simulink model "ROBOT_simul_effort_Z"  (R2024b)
settings: Solver=VariableStepAuto  StartTime=0.0  StopTime=5  RelTol=1e-3
undefined symbols (not defined in the file): a, ARRIERE_Defaut_sldprt, avant01_Defaut_sldprt, avant02_Defaut_sldprt, avant03_Defaut_sldprt, avant1_Defaut_sldprt, AXE, BASE_Defaut_sldprt, BIELLE, BIELLE_Defaut_sldprt, BRAS_Defaut_sldprt, bras_Defaut_sldprt, C_Realiste_sldprt, CABLE_Defaut_sldprt, cable_Defaut_sldprt, CACHE_Defaut_sldprt, CARTE, carte_Defaut_sldprt, CARTER, carter, CHC, CODEUR_Defaut_sldprt, cruciforme, cylindrique, deg, Drive, Fichiers, Fichiers_Matlab_sujetA, FIXATION, fixation_Defaut_sldprt, H, HEXAGONALE_Defaut_sldprt, joint_Defaut_sldprt, kg, m, M4, M4_Defaut_sldprt, manette1_Defaut_sldprt, manette2_Defaut_sldprt, MATLAB, Matlab, matlab_Defaut_sldprt, mm, modif, MOTEUR_Defaut_sldprt, N, NEZ_Defaut_sldprt, nom, palier, PARALLELOGRAMME_Defaut_sldprt, petite, plaque, rad, Ressort, Rondelle, ROTOR_Defaut_sldprt, s, SET, simple, socle_Defaut_sldprt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
libraries: sm_lib x463, fl_lib x45, nesl_utility x27, simulink x2
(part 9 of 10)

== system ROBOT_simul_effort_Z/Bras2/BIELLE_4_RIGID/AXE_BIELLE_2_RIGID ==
  ReferenceFrame : sm_lib/Frames and Transforms/Reference Frame
  Solid : sm_lib/Body Elements/File Solid  ExtGeomFileName=/MATLAB Drive/Fichiers_Matlab_sujetA/Fichiers Matlab/STL/AXE BIELLE_Defaut_sldprt.STL  UnitType=Custom  ExtGeomFileUnits=mm  StepReaderType=HEX  ExportConvexHullGeometry=off  InertiaType=Custom  BasedOnType=Density  Density=1000  DensityUnits=kg/(m^3)  Mass=0.0008880235381781051  MassUnits=kg  CenterOfMass=[0 0 0]  CenterOfMassUnits=mm  MomentsOfInertia=[0.018768660222737772 0.018768660222737772 0.0009874025874388381]  MomentsOfInertiaUnits=kg*mm^2  ProductsOfInertia=[0 0 0]  ProductsOfInertiaUnits=kg*mm^2  GraphicType=FromGeometry  MarkerShape=Sphere  MarkerSize=10  GraphicVisPropType=SimpleVisualProperties  GraphicDiffuseColor=[1 0.94901960784313721 0.90980392156862744]  GraphicOpacity=1  GraphicSpecularColor=[0.5 0.5 0.5 1.0]  GraphicAmbientColor=[0.15 0.15 0.15 1.0]  GraphicEmissiveColor=[0.0 0.0 0.0 1.0]  GraphicShininess=75  DoExposeReferenceFrame=on  SerializedFrames=<Frames/>
  F : PMIOPort  Side=Left
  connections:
  Solid/RConn1 -- ReferenceFrame/RConn1 -- F/RConn1

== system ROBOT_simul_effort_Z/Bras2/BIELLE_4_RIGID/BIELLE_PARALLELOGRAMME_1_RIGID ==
  ReferenceFrame : sm_lib/Frames and Transforms/Reference Frame
  Solid : sm_lib/Body Elements/File Solid  ExtGeomFileName=/MATLAB Drive/Fichiers_Matlab_sujetA/Fichiers Matlab/STL/BIELLE PARALLELOGRAMME_Defaut_sldprt.STL  UnitType=Custom  ExtGeomFileUnits=mm  StepReaderType=HEX  ExportConvexHullGeometry=off  InertiaType=Custom  BasedOnType=Density  Density=1000  DensityUnits=kg/(m^3)  Mass=0.0079529027635324764  MassUnits=kg  CenterOfMass=[0 3.1653377955585489 0]  CenterOfMassUnits=mm  MomentsOfInertia=[7.7987017961340088 7.8475939194203406 0.14816857834406802]  MomentsOfInertiaUnits=kg*mm^2  ProductsOfInertia=[0 0 0]  ProductsOfInertiaUnits=kg*mm^2  GraphicType=FromGeometry  MarkerShape=Sphere  MarkerSize=10  GraphicVisPropType=SimpleVisualProperties  GraphicDiffuseColor=[0.6 1.0 1.0]  GraphicOpacity=1  GraphicSpecularColor=[0.5 0.5 0.5 1.0]  GraphicAmbientColor=[0.15 0.15 0.15 1.0]  GraphicEmissiveColor=[0.0 0.0 0.0 1.0]  GraphicShininess=75  DoExposeReferenceFrame=on  SerializedFrames=<Frames/>
  F : PMIOPort  Side=Left
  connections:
  Solid/RConn1 -- ReferenceFrame/RConn1 -- F/RConn1

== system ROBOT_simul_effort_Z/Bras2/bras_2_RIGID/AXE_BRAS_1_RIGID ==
  ReferenceFrame : sm_lib/Frames and Transforms/Reference Frame
  Solid : sm_lib/Body Elements/File Solid  ExtGeomFileName=/MATLAB Drive/Fichiers_Matlab_sujetA/Fichiers Matlab/STL/AXE BRAS_Defaut_sldprt.STL  UnitType=Custom  ExtGeomFileUnits=mm  StepReaderType=HEX  ExportConvexHullGeometry=off  InertiaType=Custom  BasedOnType=Density  Density=1000  DensityUnits=kg/(m^3)  Mass=0.0015327306958088996  MassUnits=kg  CenterOfMass=[0 0 0]  CenterOfMassUnits=mm  MomentsOfInertia=[0.11359646260705632 0.11359646260705632 0.0017137152305883286]  MomentsOfInertiaUnits=kg*mm^2  ProductsOfInertia=[0 0 0]  ProductsOfInertiaUnits=kg*mm^2  GraphicType=FromGeometry  MarkerShape=Sphere  MarkerSize=10  GraphicVisPropType=SimpleVisualProperties  GraphicDiffuseColor=[0.6470588235294118 0.61960784313725492 0.58823529411764708]  GraphicOpacity=1  GraphicSpecularColor=[0.5 0.5 0.5 1.0]  GraphicAmbientColor=[0.15 0.15 0.15 1.0]  GraphicEmissiveColor=[0.0 0.0 0.0 1.0]  GraphicShininess=75  DoExposeReferenceFrame=on  SerializedFrames=<Frames/>
  F : PMIOPort  Side=Left
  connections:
  Solid/RConn1 -- ReferenceFrame/RConn1 -- F/RConn1

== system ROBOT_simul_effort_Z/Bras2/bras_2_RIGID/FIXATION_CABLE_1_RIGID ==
  ReferenceFrame : sm_lib/Frames and Transforms/Reference Frame
  Solid : sm_lib/Body Elements/File Solid  ExtGeomFileName=/MATLAB Drive/Fichiers_Matlab_sujetA/Fichiers Matlab/STL/FIXATION CABLE_Defaut_sldprt.STL  UnitType=Custom  ExtGeomFileUnits=mm  StepReaderType=HEX  ExportConvexHullGeometry=off  InertiaType=Custom  BasedOnType=Density  Density=1000  DensityUnits=kg/(m^3)  Mass=3.2000000000000007e-06  MassUnits=kg  CenterOfMass=[0 0 0.099999999999999992]  CenterOfMassUnits=mm  MomentsOfInertia=[4.2773333333333348e-06 4.2773333333333331e-06 8.5333333333333352e-06]  MomentsOfInertiaUnits=kg*mm^2  ProductsOfInertia=[0 0 0]  ProductsOfInertiaUnits=kg*mm^2  GraphicType=FromGeometry  MarkerShape=Sphere  MarkerSize=10  GraphicVisPropType=SimpleVisualProperties  GraphicDiffuseColor=[0.25098039215686274 0.25098039215686274 0.25098039215686274]  GraphicOpacity=1  GraphicSpecularColor=[0.5 0.5 0.5 1.0]  GraphicAmbientColor=[0.15 0.15 0.15 1.0]  GraphicEmissiveColor=[0.0 0.0 0.0 1.0]  GraphicShininess=75  DoExposeReferenceFrame=on  SerializedFrames=<Frames/>
  F : PMIOPort  Side=Left
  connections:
  Solid/RConn1 -- ReferenceFrame/RConn1 -- F/RConn1

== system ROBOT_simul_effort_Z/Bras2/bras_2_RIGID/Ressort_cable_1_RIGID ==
  ReferenceFrame : sm_lib/Frames and Transforms/Reference Frame
  Solid : sm_lib/Body Elements/File Solid  ExtGeomFileName=/MATLAB Drive/Fichiers_Matlab_sujetA/Fichiers Matlab/STL/Ressort cable_Defaut_sldprt.STL  UnitType=Custom  ExtGeomFileUnits=mm  StepReaderType=HEX  ExportConvexHullGeometry=off  InertiaType=Custom  BasedOnType=Density  Density=1000  DensityUnits=kg/(m^3)  Mass=0.0011765814520035881  MassUnits=kg  CenterOfMass=[0.086849073647483815 -0.00090479521327996976 6.9508776157243597]  CenterOfMassUnits=mm  MomentsOfInertia=[0.034952381374405594 0.034338972761516762 0.0097063586011258158]  MomentsOfInertiaUnits=kg*mm^2  ProductsOfInertia=[0.00037229322226744533 1.6947615167207185e-06 2.0937803976811866e-06]  ProductsOfInertiaUnits=kg*mm^2  GraphicType=FromGeometry  MarkerShape=Sphere  MarkerSize=10  GraphicVisPropType=SimpleVisualProperties  GraphicDiffuseColor=[0.6470588235294118 0.61960784313725492 0.58823529411764708]  GraphicOpacity=1  GraphicSpecularColor=[0.5 0.5 0.5 1.0]  GraphicAmbientColor=[0.15 0.15 0.15 1.0]  GraphicEmissiveColor=[0.0 0.0 0.0 1.0]  GraphicShininess=75  DoExposeReferenceFrame=on  SerializedFrames=<Frames/>
  F : PMIOPort  Side=Left
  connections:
  Solid/RConn1 -- ReferenceFrame/RConn1 -- F/RConn1

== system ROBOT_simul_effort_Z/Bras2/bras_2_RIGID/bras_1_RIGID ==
  ReferenceFrame : sm_lib/Frames and Transforms/Reference Frame
  Solid : sm_lib/Body Elements/File Solid  ExtGeomFileName=/MATLAB Drive/Fichiers_Matlab_sujetA/Fichiers Matlab/STL/bras_Defaut_sldprt.STL  UnitType=Custom  ExtGeomFileUnits=mm  StepReaderType=HEX  ExportConvexHullGeometry=off  InertiaType=Custom  BasedOnType=Density  Density=1000  DensityUnits=kg/(m^3)  Mass=0.06566875822643542  MassUnits=kg  CenterOfMass=[23.925748169887701 -4.7774352723885904 0.0071346362933715022]  CenterOfMassUnits=mm  MomentsOfInertia=[75.153076467382206 23.577652078949701 94.231108050856861]  MomentsOfInertiaUnits=kg*mm^2  ProductsOfInertia=[0.01532312637695204 0.0017211125494294708 -5.8798668472039237]  ProductsOfInertiaUnits=kg*mm^2  GraphicType=FromGeometry  MarkerShape=Sphere  MarkerSize=10  GraphicVisPropType=SimpleVisualProperties  GraphicDiffuseColor=[1.0 1.0 0.0]  GraphicOpacity=1  GraphicSpecularColor=[0.5 0.5 0.5 1.0]  GraphicAmbientColor=[0.15 0.15 0.15 1.0]  GraphicEmissiveColor=[0.0 0.0 0.0 1.0]  GraphicShininess=75  DoExposeReferenceFrame=on  SerializedFrames=<Frames/>
  F : PMIOPort  Side=Left
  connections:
  Solid/RConn1 -- ReferenceFrame/RConn1 -- F/RConn1

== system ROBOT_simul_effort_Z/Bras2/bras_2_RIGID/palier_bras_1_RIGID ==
  ReferenceFrame : sm_lib/Frames and Transforms/Reference Frame
  Solid : sm_lib/Body Elements/File Solid  ExtGeomFileName=/MATLAB Drive/Fichiers_Matlab_sujetA/Fichiers Matlab/STL/palier bras_Defaut_sldprt.STL  UnitType=Custom  ExtGeomFileUnits=mm  StepReaderType=HEX  ExportConvexHullGeometry=off  InertiaType=Custom  BasedOnType=Density  Density=1000  DensityUnits=kg/(m^3)  Mass=0.00017920168094851793  MassUnits=kg  CenterOfMass=[-178.32667601154176 39.825618202078154 -20.980989744703667]  CenterOfMassUnits=mm  MomentsOfInertia=[0.0018602253674838991 0.0012789874237151958 0.0012789874237151961]  MomentsOfInertiaUnits=kg*mm^2  ProductsOfInertia=[0 0 0]  ProductsOfInertiaUnits=kg*mm^2  GraphicType=FromGeometry  MarkerShape=Sphere  MarkerSize=10  GraphicVisPropType=SimpleVisualProperties  GraphicDiffuseColor=[1 1 1]  GraphicOpacity=1  GraphicSpecularColor=[0.5 0.5 0.5 1.0]  GraphicAmbientColor=[0.15 0.15 0.15 1.0]  GraphicEmissiveColor=[0.0 0.0 0.0 1.0]  GraphicShininess=75  DoExposeReferenceFrame=on  SerializedFrames=<Frames/>
  F : PMIOPort  Side=Left
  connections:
  Solid/RConn1 -- ReferenceFrame/RConn1 -- F/RConn1

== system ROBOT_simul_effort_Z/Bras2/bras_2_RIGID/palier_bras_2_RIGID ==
  ReferenceFrame : sm_lib/Frames and Transforms/Reference Frame
  Solid : sm_lib/Body Elements/File Solid  ExtGeomFileName=/MATLAB Drive/Fichiers_Matlab_sujetA/Fichiers Matlab/STL/palier bras_Defaut_sldprt.STL  UnitType=Custom  ExtGeomFileUnits=mm  StepReaderType=HEX  ExportConvexHullGeometry=off  InertiaType=Custom  BasedOnType=Density  Density=1000  DensityUnits=kg/(m^3)  Mass=0.00017920168094851793  MassUnits=kg  CenterOfMass=[-178.32667601154176 39.825618202078154 -20.980989744703667]  CenterOfMassUnits=mm  MomentsOfInertia=[0.0018602253674838991 0.0012789874237151958 0.0012789874237151961]  MomentsOfInertiaUnits=kg*mm^2  ProductsOfInertia=[0 0 0]  ProductsOfInertiaUnits=kg*mm^2  GraphicType=FromGeometry  MarkerShape=Sphere  MarkerSize=10  GraphicVisPropType=SimpleVisualProperties  GraphicDiffuseColor=[1 1 1]  GraphicOpacity=1  GraphicSpecularColor=[0.5 0.5 0.5 1.0]  GraphicAmbientColor=[0.15 0.15 0.15 1.0]  GraphicEmissiveColor=[0.0 0.0 0.0 1.0]  GraphicShininess=75  DoExposeReferenceFrame=on  SerializedFrames=<Frames/>
  F : PMIOPort  Side=Left
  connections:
  Solid/RConn1 -- ReferenceFrame/RConn1 -- F/RConn1

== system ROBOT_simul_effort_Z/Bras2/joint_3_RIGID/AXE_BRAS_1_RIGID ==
  ReferenceFrame : sm_lib/Frames and Transforms/Reference Frame
  Solid : sm_lib/Body Elements/File Solid  ExtGeomFileName=/MATLAB Drive/Fichiers_Matlab_sujetA/Fichiers Matlab/STL/AXE BRAS_Defaut_sldprt.STL  UnitType=Custom  ExtGeomFileUnits=mm  StepReaderType=HEX  ExportConvexHullGeometry=off  InertiaType=Custom  BasedOnType=Density  Density=1000  DensityUnits=kg/(m^3)  Mass=0.0015327306958088996  MassUnits=kg  CenterOfMass=[0 0 0]  CenterOfMassUnits=mm  MomentsOfInertia=[0.11359646260705632 0.11359646260705632 0.0017137152305883286]  MomentsOfInertiaUnits=kg*mm^2  ProductsOfInertia=[0 0 0]  ProductsOfInertiaUnits=kg*mm^2  GraphicType=FromGeometry  MarkerShape=Sphere  MarkerSize=10  GraphicVisPropType=SimpleVisualProperties  GraphicDiffuseColor=[0.6470588235294118 0.61960784313725492 0.58823529411764708]  GraphicOpacity=1  GraphicSpecularColor=[0.5 0.5 0.5 1.0]  GraphicAmbientColor=[0.15 0.15 0.15 1.0]  GraphicEmissiveColor=[0.0 0.0 0.0 1.0]  GraphicShininess=75  DoExposeReferenceFrame=on  SerializedFrames=<Frames/>
  F : PMIOPort  Side=Left
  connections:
  Solid/RConn1 -- ReferenceFrame/RConn1 -- F/RConn1

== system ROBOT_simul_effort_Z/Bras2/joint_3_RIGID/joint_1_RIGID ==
  ReferenceFrame : sm_lib/Frames and Transforms/Reference Frame
  Solid : sm_lib/Body Elements/File Solid  ExtGeomFileName=/MATLAB Drive/Fichiers_Matlab_sujetA/Fichiers Matlab/STL/joint_Defaut_sldprt.STL  UnitType=Custom  ExtGeomFileUnits=mm  StepReaderType=HEX  ExportConvexHullGeometry=off  InertiaType=Custom  BasedOnType=Density  Density=1000  DensityUnits=kg/(m^3)  Mass=0.0062454336323428689  MassUnits=kg  CenterOfMass=[-4.7519597301086606e-06 14.873568128586268 0.2827021501004604]  CenterOfMassUnits=mm  MomentsOfInertia=[0.43544209184236687 0.81590742360241675 0.91424830357082487]  MomentsOfInertiaUnits=kg*mm^2  ProductsOfInertia=[0.0068320776316595647 -4.173068650825101e-06 -7.5142319098046527e-07]  ProductsOfInertiaUnits=kg*mm^2  GraphicType=FromGeometry  MarkerShape=Sphere  MarkerSize=10  GraphicVisPropType=SimpleVisualProperties  GraphicDiffuseColor=[1 1 1]  GraphicOpacity=1  GraphicSpecularColor=[0.5 0.5 0.5 1.0]  GraphicAmbientColor=[0.15 0.15 0.15 1.0]  GraphicEmissiveColor=[0.0 0.0 0.0 1.0]  GraphicShininess=75  DoExposeReferenceFrame=on  SerializedFrames=<Frames/>
  F : PMIOPort  Side=Left
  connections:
  Solid/RConn1 -- ReferenceFrame/RConn1 -- F/RConn1

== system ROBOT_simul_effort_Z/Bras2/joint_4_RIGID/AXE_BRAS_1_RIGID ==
  ReferenceFrame : sm_lib/Frames and Transforms/Reference Frame
  Solid : sm_lib/Body Elements/File Solid  ExtGeomFileName=/MATLAB Drive/Fichiers_Matlab_sujetA/Fichiers Matlab/STL/AXE BRAS_Defaut_sldprt.STL  UnitType=Custom  ExtGeomFileUnits=mm  StepReaderType=HEX  ExportConvexHullGeometry=off  InertiaType=Custom  BasedOnType=Density  Density=1000  DensityUnits=kg/(m^3)  Mass=0.0015327306958088996  MassUnits=kg  CenterOfMass=[0 0 0]  CenterOfMassUnits=mm  MomentsOfInertia=[0.11359646260705632 0.11359646260705632 0.0017137152305883286]  MomentsOfInertiaUnits=kg*mm^2  ProductsOfInertia=[0 0 0]  ProductsOfInertiaUnits=kg*mm^2  GraphicType=FromGeometry  MarkerShape=Sphere  MarkerSize=10  GraphicVisPropType=SimpleVisualProperties  GraphicDiffuseColor=[0.6470588235294118 0.61960784313725492 0.58823529411764708]  GraphicOpacity=1  GraphicSpecularColor=[0.5 0.5 0.5 1.0]  GraphicAmbientColor=[0.15 0.15 0.15 1.0]  GraphicEmissiveColor=[0.0 0.0 0.0 1.0]  GraphicShininess=75  DoExposeReferenceFrame=on  SerializedFrames=<Frames/>
  F : PMIOPort  Side=Left
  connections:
  Solid/RConn1 -- ReferenceFrame/RConn1 -- F/RConn1

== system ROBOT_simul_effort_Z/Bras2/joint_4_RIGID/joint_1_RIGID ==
  ReferenceFrame : sm_lib/Frames and Transforms/Reference Frame
  Solid : sm_lib/Body Elements/File Solid  ExtGeomFileName=/MATLAB Drive/Fichiers_Matlab_sujetA/Fichiers Matlab/STL/joint_Defaut_sldprt.STL  UnitType=Custom  ExtGeomFileUnits=mm  StepReaderType=HEX  ExportConvexHullGeometry=off  InertiaType=Custom  BasedOnType=Density  Density=1000  DensityUnits=kg/(m^3)  Mass=0.0062454336323428689  MassUnits=kg  CenterOfMass=[-4.7519597301086606e-06 14.873568128586268 0.2827021501004604]  CenterOfMassUnits=mm  MomentsOfInertia=[0.43544209184236687 0.81590742360241675 0.91424830357082487]  MomentsOfInertiaUnits=kg*mm^2  ProductsOfInertia=[0.0068320776316595647 -4.173068650825101e-06 -7.5142319098046527e-07]  ProductsOfInertiaUnits=kg*mm^2  GraphicType=FromGeometry  MarkerShape=Sphere  MarkerSize=10  GraphicVisPropType=SimpleVisualProperties  GraphicDiffuseColor=[1 1 1]  GraphicOpacity=1  GraphicSpecularColor=[0.5 0.5 0.5 1.0]  GraphicAmbientColor=[0.15 0.15 0.15 1.0]  GraphicEmissiveColor=[0.0 0.0 0.0 1.0]  GraphicShininess=75  DoExposeReferenceFrame=on  SerializedFrames=<Frames/>
  F : PMIOPort  Side=Left
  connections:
  Solid/RConn1 -- ReferenceFrame/RConn1 -- F/RConn1

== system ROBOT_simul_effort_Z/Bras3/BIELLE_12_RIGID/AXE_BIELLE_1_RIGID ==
  ReferenceFrame : sm_lib/Frames and Transforms/Reference Frame
  Solid : sm_lib/Body Elements/File Solid  ExtGeomFileName=/MATLAB Drive/Fichiers_Matlab_sujetA/Fichiers Matlab/STL/AXE BIELLE_Defaut_sldprt.STL  UnitType=Custom  ExtGeomFileUnits=mm  StepReaderType=HEX  ExportConvexHullGeometry=off  InertiaType=Custom  BasedOnType=Density  Density=1000  DensityUnits=kg/(m^3)  Mass=0.0008880235381781051  MassUnits=kg  CenterOfMass=[0 0 0]  CenterOfMassUnits=mm  MomentsOfInertia=[0.018768660222737772 0.018768660222737772 0.0009874025874388381]  MomentsOfInertiaUnits=kg*mm^2  ProductsOfInertia=[0 0 0]  ProductsOfInertiaUnits=kg*mm^2  GraphicType=FromGeometry  MarkerShape=Sphere  MarkerSize=10  GraphicVisPropType=SimpleVisualProperties  GraphicDiffuseColor=[1 0.94901960784313721 0.90980392156862744]  GraphicOpacity=1  GraphicSpecularColor=[0.5 0.5 0.5 1.0]  GraphicAmbientColor=[0.15 0.15 0.15 1.0]  GraphicEmissiveColor=[0.0 0.0 0.0 1.0]  GraphicShininess=75  DoExposeReferenceFrame=on  SerializedFrames=<Frames/>
  F : PMIOPort  Side=Left
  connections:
  Solid/RConn1 -- ReferenceFrame/RConn1 -- F/RConn1

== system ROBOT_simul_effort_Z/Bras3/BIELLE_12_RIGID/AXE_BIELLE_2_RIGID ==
  ReferenceFrame : sm_lib/Frames and Transforms/Reference Frame
  Solid : sm_lib/Body Elements/File Solid  ExtGeomFileName=/MATLAB Drive/Fichiers_Matlab_sujetA/Fichiers Matlab/STL/AXE BIELLE_Defaut_sldprt.STL  UnitType=Custom  ExtGeomFileUnits=mm  StepReaderType=HEX  ExportConvexHullGeometry=off  InertiaType=Custom  BasedOnType=Density  Density=1000  DensityUnits=kg/(m^3)  Mass=0.0008880235381781051  MassUnits=kg  CenterOfMass=[0 0 0]  CenterOfMassUnits=mm  MomentsOfInertia=[0.018768660222737772 0.018768660222737772 0.0009874025874388381]  MomentsOfInertiaUnits=kg*mm^2  ProductsOfInertia=[0 0 0]  ProductsOfInertiaUnits=kg*mm^2  GraphicType=FromGeometry  MarkerShape=Sphere  MarkerSize=10  GraphicVisPropType=SimpleVisualProperties  GraphicDiffuseColor=[1 0.94901960784313721 0.90980392156862744]  GraphicOpacity=1  GraphicSpecularColor=[0.5 0.5 0.5 1.0]  GraphicAmbientColor=[0.15 0.15 0.15 1.0]  GraphicEmissiveColor=[0.0 0.0 0.0 1.0]  GraphicShininess=75  DoExposeReferenceFrame=on  SerializedFrames=<Frames/>
  F : PMIOPort  Side=Left
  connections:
  Solid/RConn1 -- ReferenceFrame/RConn1 -- F/RConn1

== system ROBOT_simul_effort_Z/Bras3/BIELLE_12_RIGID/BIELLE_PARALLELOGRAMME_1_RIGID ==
  ReferenceFrame : sm_lib/Frames and Transforms/Reference Frame
  Solid : sm_lib/Body Elements/File Solid  ExtGeomFileName=/MATLAB Drive/Fichiers_Matlab_sujetA/Fichiers Matlab/STL/BIELLE PARALLELOGRAMME_Defaut_sldprt.STL  UnitType=Custom  ExtGeomFileUnits=mm  StepReaderType=HEX  ExportConvexHullGeometry=off  InertiaType=Custom  BasedOnType=Density  Density=1000  DensityUnits=kg/(m^3)  Mass=0.0079529027635324764  MassUnits=kg  CenterOfMass=[0 3.1653377955585489 0]  CenterOfMassUnits=mm  MomentsOfInertia=[7.7987017961340088 7.8475939194203406 0.14816857834406802]  MomentsOfInertiaUnits=kg*mm^2  ProductsOfInertia=[0 0 0]  ProductsOfInertiaUnits=kg*mm^2  GraphicType=FromGeometry  MarkerShape=Sphere  MarkerSize=10  GraphicVisPropType=SimpleVisualProperties  GraphicDiffuseColor=[0.6 1.0 1.0]  GraphicOpacity=1  GraphicSpecularColor=[0.5 0.5 0.5 1.0]  GraphicAmbientColor=[0.15 0.15 0.15 1.0]  GraphicEmissiveColor=[0.0 0.0 0.0 1.0]  GraphicShininess=75  DoExposeReferenceFrame=on  SerializedFrames=<Frames/>
  F : PMIOPort  Side=Left
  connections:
  Solid/RConn1 -- ReferenceFrame/RConn1 -- F/RConn1

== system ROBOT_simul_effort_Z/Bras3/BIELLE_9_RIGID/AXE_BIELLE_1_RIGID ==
  ReferenceFrame : sm_lib/Frames and Transforms/Reference Frame
  Solid : sm_lib/Body Elements/File Solid  ExtGeomFileName=/MATLAB Drive/Fichiers_Matlab_sujetA/Fichiers Matlab/STL/AXE BIELLE_Defaut_sldprt.STL  UnitType=Custom  ExtGeomFileUnits=mm  StepReaderType=HEX  ExportConvexHullGeometry=off  InertiaType=Custom  BasedOnType=Density  Density=1000  DensityUnits=kg/(m^3)  Mass=0.0008880235381781051  MassUnits=kg  CenterOfMass=[0 0 0]  CenterOfMassUnits=mm  MomentsOfInertia=[0.018768660222737772 0.018768660222737772 0.0009874025874388381]  MomentsOfInertiaUnits=kg*mm^2  ProductsOfInertia=[0 0 0]  ProductsOfInertiaUnits=kg*mm^2  GraphicType=FromGeometry  MarkerShape=Sphere  MarkerSize=10  GraphicVisPropType=SimpleVisualProperties  GraphicDiffuseColor=[1 0.94901960784313721 0.90980392156862744]  GraphicOpacity=1  GraphicSpecularColor=[0.5 0.5 0.5 1.0]  GraphicAmbientColor=[0.15 0.15 0.15 1.0]  GraphicEmissiveColor=[0.0 0.0 0.0 1.0]  GraphicShininess=75  DoExposeReferenceFrame=on  SerializedFrames=<Frames/>
  F : PMIOPort  Side=Left
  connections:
  Solid/RConn1 -- ReferenceFrame/RConn1 -- F/RConn1

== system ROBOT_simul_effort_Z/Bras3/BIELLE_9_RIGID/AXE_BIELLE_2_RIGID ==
  ReferenceFrame : sm_lib/Frames and Transforms/Reference Frame
  Solid : sm_lib/Body Elements/File Solid  ExtGeomFileName=/MATLAB Drive/Fichiers_Matlab_sujetA/Fichiers Matlab/STL/AXE BIELLE_Defaut_sldprt.STL  UnitType=Custom  ExtGeomFileUnits=mm  StepReaderType=HEX  ExportConvexHullGeometry=off  InertiaType=Custom  BasedOnType=Density  Density=1000  DensityUnits=kg/(m^3)  Mass=0.0008880235381781051  MassUnits=kg  CenterOfMass=[0 0 0]  CenterOfMassUnits=mm  MomentsOfInertia=[0.018768660222737772 0.018768660222737772 0.0009874025874388381]  MomentsOfInertiaUnits=kg*mm^2  ProductsOfInertia=[0 0 0]  ProductsOfInertiaUnits=kg*mm^2  GraphicType=FromGeometry  MarkerShape=Sphere  MarkerSize=10  GraphicVisPropType=SimpleVisualProperties  GraphicDiffuseColor=[1 0.94901960784313721 0.90980392156862744]  GraphicOpacity=1  GraphicSpecularColor=[0.5 0.5 0.5 1.0]  GraphicAmbientColor=[0.15 0.15 0.15 1.0]  GraphicEmissiveColor=[0.0 0.0 0.0 1.0]  GraphicShininess=75  DoExposeReferenceFrame=on  SerializedFrames=<Frames/>
  F : PMIOPort  Side=Left
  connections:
  Solid/RConn1 -- ReferenceFrame/RConn1 -- F/RConn1

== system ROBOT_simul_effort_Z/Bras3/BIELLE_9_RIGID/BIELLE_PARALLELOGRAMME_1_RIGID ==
  ReferenceFrame : sm_lib/Frames and Transforms/Reference Frame
  Solid : sm_lib/Body Elements/File Solid  ExtGeomFileName=/MATLAB Drive/Fichiers_Matlab_sujetA/Fichiers Matlab/STL/BIELLE PARALLELOGRAMME_Defaut_sldprt.STL  UnitType=Custom  ExtGeomFileUnits=mm  StepReaderType=HEX  ExportConvexHullGeometry=off  InertiaType=Custom  BasedOnType=Density  Density=1000  DensityUnits=kg/(m^3)  Mass=0.0079529027635324764  MassUnits=kg  CenterOfMass=[0 3.1653377955585489 0]  CenterOfMassUnits=mm  MomentsOfInertia=[7.7987017961340088 7.8475939194203406 0.14816857834406802]  MomentsOfInertiaUnits=kg*mm^2  ProductsOfInertia=[0 0 0]  ProductsOfInertiaUnits=kg*mm^2  GraphicType=FromGeometry  MarkerShape=Sphere  MarkerSize=10  GraphicVisPropType=SimpleVisualProperties  GraphicDiffuseColor=[0.6 1.0 1.0]  GraphicOpacity=1  GraphicSpecularColor=[0.5 0.5 0.5 1.0]  GraphicAmbientColor=[0.15 0.15 0.15 1.0]  GraphicEmissiveColor=[0.0 0.0 0.0 1.0]  GraphicShininess=75  DoExposeReferenceFrame=on  SerializedFrames=<Frames/>
  F : PMIOPort  Side=Left
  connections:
  Solid/RConn1 -- ReferenceFrame/RConn1 -- F/RConn1

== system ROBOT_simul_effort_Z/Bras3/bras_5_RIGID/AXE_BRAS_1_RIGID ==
  ReferenceFrame : sm_lib/Frames and Transforms/Reference Frame
  Solid : sm_lib/Body Elements/File Solid  ExtGeomFileName=/MATLAB Drive/Fichiers_Matlab_sujetA/Fichiers Matlab/STL/AXE BRAS_Defaut_sldprt.STL  UnitType=Custom  ExtGeomFileUnits=mm  StepReaderType=HEX  ExportConvexHullGeometry=off  InertiaType=Custom  BasedOnType=Density  Density=1000  DensityUnits=kg/(m^3)  Mass=0.0015327306958088996  MassUnits=kg  CenterOfMass=[0 0 0]  CenterOfMassUnits=mm  MomentsOfInertia=[0.11359646260705632 0.11359646260705632 0.0017137152305883286]  MomentsOfInertiaUnits=kg*mm^2  ProductsOfInertia=[0 0 0]  ProductsOfInertiaUnits=kg*mm^2  GraphicType=FromGeometry  MarkerShape=Sphere  MarkerSize=10  GraphicVisPropType=SimpleVisualProperties  GraphicDiffuseColor=[0.6470588235294118 0.61960784313725492 0.58823529411764708]  GraphicOpacity=1  GraphicSpecularColor=[0.5 0.5 0.5 1.0]  GraphicAmbientColor=[0.15 0.15 0.15 1.0]  GraphicEmissiveColor=[0.0 0.0 0.0 1.0]  GraphicShininess=75  DoExposeReferenceFrame=on  SerializedFrames=<Frames/>
  F : PMIOPort  Side=Left
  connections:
  Solid/RConn1 -- ReferenceFrame/RConn1 -- F/RConn1

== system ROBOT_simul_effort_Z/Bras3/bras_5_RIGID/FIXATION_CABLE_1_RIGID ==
  ReferenceFrame : sm_lib/Frames and Transforms/Reference Frame
  Solid : sm_lib/Body Elements/File Solid  ExtGeomFileName=/MATLAB Drive/Fichiers_Matlab_sujetA/Fichiers Matlab/STL/FIXATION CABLE_Defaut_sldprt.STL  UnitType=Custom  ExtGeomFileUnits=mm  StepReaderType=HEX  ExportConvexHullGeometry=off  InertiaType=Custom  BasedOnType=Density  Density=1000  DensityUnits=kg/(m^3)  Mass=3.2000000000000007e-06  MassUnits=kg  CenterOfMass=[0 0 0.099999999999999992]  CenterOfMassUnits=mm  MomentsOfInertia=[4.2773333333333348e-06 4.2773333333333331e-06 8.5333333333333352e-06]  MomentsOfInertiaUnits=kg*mm^2  ProductsOfInertia=[0 0 0]  ProductsOfInertiaUnits=kg*mm^2  GraphicType=FromGeometry  MarkerShape=Sphere  MarkerSize=10  GraphicVisPropType=SimpleVisualProperties  GraphicDiffuseColor=[0.25098039215686274 0.25098039215686274 0.25098039215686274]  GraphicOpacity=1  GraphicSpecularColor=[0.5 0.5 0.5 1.0]  GraphicAmbientColor=[0.15 0.15 0.15 1.0]  GraphicEmissiveColor=[0.0 0.0 0.0 1.0]  GraphicShininess=75  DoExposeReferenceFrame=on  SerializedFrames=<Frames/>
  F : PMIOPort  Side=Left
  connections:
  Solid/RConn1 -- ReferenceFrame/RConn1 -- F/RConn1

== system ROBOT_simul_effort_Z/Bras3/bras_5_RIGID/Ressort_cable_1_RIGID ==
  ReferenceFrame : sm_lib/Frames and Transforms/Reference Frame
  Solid : sm_lib/Body Elements/File Solid  ExtGeomFileName=/MATLAB Drive/Fichiers_Matlab_sujetA/Fichiers Matlab/STL/Ressort cable_Defaut_sldprt.STL  UnitType=Custom  ExtGeomFileUnits=mm  StepReaderType=HEX  ExportConvexHullGeometry=off  InertiaType=Custom  BasedOnType=Density  Density=1000  DensityUnits=kg/(m^3)  Mass=0.0011765814520035881  MassUnits=kg  CenterOfMass=[0.086849073647483815 -0.00090479521327996976 6.9508776157243597]  CenterOfMassUnits=mm  MomentsOfInertia=[0.034952381374405594 0.034338972761516762 0.0097063586011258158]  MomentsOfInertiaUnits=kg*mm^2  ProductsOfInertia=[0.00037229322226744533 1.6947615167207185e-06 2.0937803976811866e-06]  ProductsOfInertiaUnits=kg*mm^2  GraphicType=FromGeometry  MarkerShape=Sphere  MarkerSize=10  GraphicVisPropType=SimpleVisualProperties  GraphicDiffuseColor=[0.6470588235294118 0.61960784313725492 0.58823529411764708]  GraphicOpacity=1  GraphicSpecularColor=[0.5 0.5 0.5 1.0]  GraphicAmbientColor=[0.15 0.15 0.15 1.0]  GraphicEmissiveColor=[0.0 0.0 0.0 1.0]  GraphicShininess=75  DoExposeReferenceFrame=on  SerializedFrames=<Frames/>
  F : PMIOPort  Side=Left
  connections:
  Solid/RConn1 -- ReferenceFrame/RConn1 -- F/RConn1

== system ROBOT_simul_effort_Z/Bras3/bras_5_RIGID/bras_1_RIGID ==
  ReferenceFrame : sm_lib/Frames and Transforms/Reference Frame
  Solid : sm_lib/Body Elements/File Solid  ExtGeomFileName=/MATLAB Drive/Fichiers_Matlab_sujetA/Fichiers Matlab/STL/bras_Defaut_sldprt.STL  UnitType=Custom  ExtGeomFileUnits=mm  StepReaderType=HEX  ExportConvexHullGeometry=off  InertiaType=Custom  BasedOnType=Density  Density=1000  DensityUnits=kg/(m^3)  Mass=0.06566875822643542  MassUnits=kg  CenterOfMass=[23.925748169887701 -4.7774352723885904 0.0071346362933715022]  CenterOfMassUnits=mm  MomentsOfInertia=[75.153076467382206 23.577652078949701 94.231108050856861]  MomentsOfInertiaUnits=kg*mm^2  ProductsOfInertia=[0.01532312637695204 0.0017211125494294708 -5.8798668472039237]  ProductsOfInertiaUnits=kg*mm^2  GraphicType=FromGeometry  MarkerShape=Sphere  MarkerSize=10  GraphicVisPropType=SimpleVisualProperties  GraphicDiffuseColor=[1.0 1.0 0.0]  GraphicOpacity=1  GraphicSpecularColor=[0.5 0.5 0.5 1.0]  GraphicAmbientColor=[0.15 0.15 0.15 1.0]  GraphicEmissiveColor=[0.0 0.0 0.0 1.0]  GraphicShininess=75  DoExposeReferenceFrame=on  SerializedFrames=<Frames/>
  F : PMIOPort  Side=Left
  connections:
  Solid/RConn1 -- ReferenceFrame/RConn1 -- F/RConn1

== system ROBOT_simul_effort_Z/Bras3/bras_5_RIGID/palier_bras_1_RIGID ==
  ReferenceFrame : sm_lib/Frames and Transforms/Reference Frame
  Solid : sm_lib/Body Elements/File Solid  ExtGeomFileName=/MATLAB Drive/Fichiers_Matlab_sujetA/Fichiers Matlab/STL/palier bras_Defaut_sldprt.STL  UnitType=Custom  ExtGeomFileUnits=mm  StepReaderType=HEX  ExportConvexHullGeometry=off  InertiaType=Custom  BasedOnType=Density  Density=1000  DensityUnits=kg/(m^3)  Mass=0.00017920168094851793  MassUnits=kg  CenterOfMass=[-178.32667601154176 39.825618202078154 -20.980989744703667]  CenterOfMassUnits=mm  MomentsOfInertia=[0.0018602253674838991 0.0012789874237151958 0.0012789874237151961]  MomentsOfInertiaUnits=kg*mm^2  ProductsOfInertia=[0 0 0]  ProductsOfInertiaUnits=kg*mm^2  GraphicType=FromGeometry  MarkerShape=Sphere  MarkerSize=10  GraphicVisPropType=SimpleVisualProperties  GraphicDiffuseColor=[1 1 1]  GraphicOpacity=1  GraphicSpecularColor=[0.5 0.5 0.5 1.0]  GraphicAmbientColor=[0.15 0.15 0.15 1.0]  GraphicEmissiveColor=[0.0 0.0 0.0 1.0]  GraphicShininess=75  DoExposeReferenceFrame=on  SerializedFrames=<Frames/>
  F : PMIOPort  Side=Left
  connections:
  Solid/RConn1 -- ReferenceFrame/RConn1 -- F/RConn1

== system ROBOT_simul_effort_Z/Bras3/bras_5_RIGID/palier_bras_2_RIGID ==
  ReferenceFrame : sm_lib/Frames and Transforms/Reference Frame
  Solid : sm_lib/Body Elements/File Solid  ExtGeomFileName=/MATLAB Drive/Fichiers_Matlab_sujetA/Fichiers Matlab/STL/palier bras_Defaut_sldprt.STL  UnitType=Custom  ExtGeomFileUnits=mm  StepReaderType=HEX  ExportConvexHullGeometry=off  InertiaType=Custom  BasedOnType=Density  Density=1000  DensityUnits=kg/(m^3)  Mass=0.00017920168094851793  MassUnits=kg  CenterOfMass=[-178.32667601154176 39.825618202078154 -20.980989744703667]  CenterOfMassUnits=mm  MomentsOfInertia=[0.0018602253674838991 0.0012789874237151958 0.0012789874237151961]  MomentsOfInertiaUnits=kg*mm^2  ProductsOfInertia=[0 0 0]  ProductsOfInertiaUnits=kg*mm^2  GraphicType=FromGeometry  MarkerShape=Sphere  MarkerSize=10  GraphicVisPropType=SimpleVisualProperties  GraphicDiffuseColor=[1 1 1]  GraphicOpacity=1  GraphicSpecularColor=[0.5 0.5 0.5 1.0]  GraphicAmbientColor=[0.15 0.15 0.15 1.0]  GraphicEmissiveColor=[0.0 0.0 0.0 1.0]  GraphicShininess=75  DoExposeReferenceFrame=on  SerializedFrames=<Frames/>
  F : PMIOPort  Side=Left
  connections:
  Solid/RConn1 -- ReferenceFrame/RConn1 -- F/RConn1

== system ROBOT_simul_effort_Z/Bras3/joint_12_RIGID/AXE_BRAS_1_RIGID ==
  ReferenceFrame : sm_lib/Frames and Transforms/Reference Frame
  Solid : sm_lib/Body Elements/File Solid  ExtGeomFileName=/MATLAB Drive/Fichiers_Matlab_sujetA/Fichiers Matlab/STL/AXE BRAS_Defaut_sldprt.STL  UnitType=Custom  ExtGeomFileUnits=mm  StepReaderType=HEX  ExportConvexHullGeometry=off  InertiaType=Custom  BasedOnType=Density  Density=1000  DensityUnits=kg/(m^3)  Mass=0.0015327306958088996  MassUnits=kg  CenterOfMass=[0 0 0]  CenterOfMassUnits=mm  MomentsOfInertia=[0.11359646260705632 0.11359646260705632 0.0017137152305883286]  MomentsOfInertiaUnits=kg*mm^2  ProductsOfInertia=[0 0 0]  ProductsOfInertiaUnits=kg*mm^2  GraphicType=FromGeometry  MarkerShape=Sphere  MarkerSize=10  GraphicVisPropType=SimpleVisualProperties  GraphicDiffuseColor=[0.6470588235294118 0.61960784313725492 0.58823529411764708]  GraphicOpacity=1  GraphicSpecularColor=[0.5 0.5 0.5 1.0]  GraphicAmbientColor=[0.15 0.15 0.15 1.0]  GraphicEmissiveColor=[0.0 0.0 0.0 1.0]  GraphicShininess=75  DoExposeReferenceFrame=on  SerializedFrames=<Frames/>
  F : PMIOPort  Side=Left
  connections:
  Solid/RConn1 -- ReferenceFrame/RConn1 -- F/RConn1

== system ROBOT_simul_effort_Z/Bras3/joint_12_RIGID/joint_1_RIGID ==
  ReferenceFrame : sm_lib/Frames and Transforms/Reference Frame
  Solid : sm_lib/Body Elements/File Solid  ExtGeomFileName=/MATLAB Drive/Fichiers_Matlab_sujetA/Fichiers Matlab/STL/joint_Defaut_sldprt.STL  UnitType=Custom  ExtGeomFileUnits=mm  StepReaderType=HEX  ExportConvexHullGeometry=off  InertiaType=Custom  BasedOnType=Density  Density=1000  DensityUnits=kg/(m^3)  Mass=0.0062454336323428689  MassUnits=kg  CenterOfMass=[-4.7519597301086606e-06 14.873568128586268 0.2827021501004604]  CenterOfMassUnits=mm  MomentsOfInertia=[0.43544209184236687 0.81590742360241675 0.91424830357082487]  MomentsOfInertiaUnits=kg*mm^2  ProductsOfInertia=[0.0068320776316595647 -4.173068650825101e-06 -7.5142319098046527e-07]  ProductsOfInertiaUnits=kg*mm^2  GraphicType=FromGeometry  MarkerShape=Sphere  MarkerSize=10  GraphicVisPropType=SimpleVisualProperties  GraphicDiffuseColor=[1 1 1]  GraphicOpacity=1  GraphicSpecularColor=[0.5 0.5 0.5 1.0]  GraphicAmbientColor=[0.15 0.15 0.15 1.0]  GraphicEmissiveColor=[0.0 0.0 0.0 1.0]  GraphicShininess=75  DoExposeReferenceFrame=on  SerializedFrames=<Frames/>
  F : PMIOPort  Side=Left
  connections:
  Solid/RConn1 -- ReferenceFrame/RConn1 -- F/RConn1

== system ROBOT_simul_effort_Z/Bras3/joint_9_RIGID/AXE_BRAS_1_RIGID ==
  ReferenceFrame : sm_lib/Frames and Transforms/Reference Frame
  Solid : sm_lib/Body Elements/File Solid  ExtGeomFileName=/MATLAB Drive/Fichiers_Matlab_sujetA/Fichiers Matlab/STL/AXE BRAS_Defaut_sldprt.STL  UnitType=Custom  ExtGeomFileUnits=mm  StepReaderType=HEX  ExportConvexHullGeometry=off  InertiaType=Custom  BasedOnType=Density  Density=1000  DensityUnits=kg/(m^3)  Mass=0.0015327306958088996  MassUnits=kg  CenterOfMass=[0 0 0]  CenterOfMassUnits=mm  MomentsOfInertia=[0.11359646260705632 0.11359646260705632 0.0017137152305883286]  MomentsOfInertiaUnits=kg*mm^2  ProductsOfInertia=[0 0 0]  ProductsOfInertiaUnits=kg*mm^2  GraphicType=FromGeometry  MarkerShape=Sphere  MarkerSize=10  GraphicVisPropType=SimpleVisualProperties  GraphicDiffuseColor=[0.6470588235294118 0.61960784313725492 0.58823529411764708]  GraphicOpacity=1  GraphicSpecularColor=[0.5 0.5 0.5 1.0]  GraphicAmbientColor=[0.15 0.15 0.15 1.0]  GraphicEmissiveColor=[0.0 0.0 0.0 1.0]  GraphicShininess=75  DoExposeReferenceFrame=on  SerializedFrames=<Frames/>
  F : PMIOPort  Side=Left
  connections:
  Solid/RConn1 -- ReferenceFrame/RConn1 -- F/RConn1

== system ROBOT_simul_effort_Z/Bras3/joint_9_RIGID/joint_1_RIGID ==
  ReferenceFrame : sm_lib/Frames and Transforms/Reference Frame
  Solid : sm_lib/Body Elements/File Solid  ExtGeomFileName=/MATLAB Drive/Fichiers_Matlab_sujetA/Fichiers Matlab/STL/joint_Defaut_sldprt.STL  UnitType=Custom  ExtGeomFileUnits=mm  StepReaderType=HEX  ExportConvexHullGeometry=off  InertiaType=Custom  BasedOnType=Density  Density=1000  DensityUnits=kg/(m^3)  Mass=0.0062454336323428689  MassUnits=kg  CenterOfMass=[-4.7519597301086606e-06 14.873568128586268 0.2827021501004604]  CenterOfMassUnits=mm  MomentsOfInertia=[0.43544209184236687 0.81590742360241675 0.91424830357082487]  MomentsOfInertiaUnits=kg*mm^2  ProductsOfInertia=[0.0068320776316595647 -4.173068650825101e-06 -7.5142319098046527e-07]  ProductsOfInertiaUnits=kg*mm^2  GraphicType=FromGeometry  MarkerShape=Sphere  MarkerSize=10  GraphicVisPropType=SimpleVisualProperties  GraphicDiffuseColor=[1 1 1]  GraphicOpacity=1  GraphicSpecularColor=[0.5 0.5 0.5 1.0]  GraphicAmbientColor=[0.15 0.15 0.15 1.0]  GraphicEmissiveColor=[0.0 0.0 0.0 1.0]  GraphicShininess=75  DoExposeReferenceFrame=on  SerializedFrames=<Frames/>
  F : PMIOPort  Side=Left
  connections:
  Solid/RConn1 -- ReferenceFrame/RConn1 -- F/RConn1

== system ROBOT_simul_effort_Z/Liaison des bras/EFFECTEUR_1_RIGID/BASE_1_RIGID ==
  ReferenceFrame : sm_lib/Frames and Transforms/Reference Frame
  Solid : sm_lib/Body Elements/File Solid  ExtGeomFileName=/MATLAB Drive/Fichiers_Matlab_sujetA/Fichiers Matlab/STL/BASE_Defaut_sldprt.STL  UnitType=Custom  ExtGeomFileUnits=mm  StepReaderType=HEX  ExportConvexHullGeometry=off  InertiaType=Custom  BasedOnType=Density  Density=1000  DensityUnits=kg/(m^3)  Mass=0.028238598075005058  MassUnits=kg  CenterOfMass=[-0.50940754911928388 -1.6318221689243708 -4.5607511741024656]  CenterOfMassUnits=mm  MomentsOfInertia=[8.5842414198569479 7.5819347196129669 14.129620619032369]  MomentsOfInertiaUnits=kg*mm^2  ProductsOfInertia=[-0.29549774773685261 -0.082418003511546406 -0.14811223553088118]  ProductsOfInertiaUnits=kg*mm^2  GraphicType=FromGeometry  MarkerShape=Sphere  MarkerSize=10  GraphicVisPropType=SimpleVisualProperties  GraphicDiffuseColor=[1.0 1.0 1.0]  GraphicOpacity=1  GraphicSpecularColor=[0.5 0.5 0.5 1.0]  GraphicAmbientColor=[0.15 0.15 0.15 1.0]  GraphicEmissiveColor=[0.0 0.0 0.0 1.0]  GraphicShininess=75  DoExposeReferenceFrame=on  SerializedFrames=<Frames/>
  F : PMIOPort  Side=Left
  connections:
  Solid/RConn1 -- ReferenceFrame/RConn1 -- F/RConn1

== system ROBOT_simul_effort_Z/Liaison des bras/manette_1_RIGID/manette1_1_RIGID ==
  ReferenceFrame : sm_lib/Frames and Transforms/Reference Frame
  Solid : sm_lib/Body Elements/File Solid  ExtGeomFileName=/MATLAB Drive/Fichiers_Matlab_sujetA/Fichiers Matlab/STL/manette1_Defaut_sldprt.STL  UnitType=Custom  ExtGeomFileUnits=mm  StepReaderType=HEX  ExportConvexHullGeometry=off  InertiaType=Custom  BasedOnType=Density  Density=1000  DensityUnits=kg/(m^3)  Mass=0.021495200046783486  MassUnits=kg  CenterOfMass=[-1.4897475291331288 1.1324325333899619 3.6124835128376875]  CenterOfMassUnits=mm  MomentsOfInertia=[5.4184345928892519 5.4614392106741905 10.048915162120133]  MomentsOfInertiaUnits=kg*mm^2  ProductsOfInertia=[-0.010452851512005331 -0.0018797921399214363 0.024517118393881449]  ProductsOfInertiaUnits=kg*mm^2  GraphicType=FromGeometry  MarkerShape=Sphere  MarkerSize=10  GraphicVisPropType=SimpleVisualProperties  GraphicDiffuseColor=[0.8 0.8 0.8]  GraphicOpacity=1  GraphicSpecularColor=[0.5 0.5 0.5 1.0]  GraphicAmbientColor=[0.15 0.15 0.15 1.0]  GraphicEmissiveColor=[0.0 0.0 0.0 1.0]  GraphicShininess=75  DoExposeReferenceFrame=on  SerializedFrames=<Frames/>
  F : PMIOPort  Side=Left
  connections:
  Solid/RConn1 -- ReferenceFrame/RConn1 -- F/RConn1

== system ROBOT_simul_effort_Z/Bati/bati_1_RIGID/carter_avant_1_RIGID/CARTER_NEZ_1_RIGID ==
  ReferenceFrame : sm_lib/Frames and Transforms/Reference Frame
  Solid : sm_lib/Body Elements/File Solid  ExtGeomFileName=/MATLAB Drive/Fichiers_Matlab_sujetA/Fichiers Matlab/STL/CARTER NEZ_Defaut_sldprt.STL  UnitType=Custom  ExtGeomFileUnits=mm  StepReaderType=HEX  ExportConvexHullGeometry=off  InertiaType=Custom  BasedOnType=Density  Density=1000  DensityUnits=kg/(m^3)  Mass=0.023684568109850399  MassUnits=kg  CenterOfMass=[17.102684932647009 114.0476537917955 1.3404873933864438]  CenterOfMassUnits=mm  MomentsOfInertia=[16.43130676036915 32.571595129912247 16.431105891514132]  MomentsOfInertiaUnits=kg*mm^2  ProductsOfInertia=[-3.788014627850142e-05 -4.8452777139477129e-05 -5.4026210558728518e-06]  ProductsOfInertiaUnits=kg*mm^2  GraphicType=FromGeometry  MarkerShape=Sphere  MarkerSize=10  GraphicVisPropType=SimpleVisualProperties  GraphicDiffuseColor=[0.75294117647058822 0.75294117647058822 0.75294117647058822]  GraphicOpacity=1  GraphicSpecularColor=[0.5 0.5 0.5 1.0]  GraphicAmbientColor=[0.15 0.15 0.15 1.0]  GraphicEmissiveColor=[0.0 0.0 0.0 1.0]  GraphicShininess=75  DoExposeReferenceFrame=on  SerializedFrames=<Frames/>
  F : PMIOPort  Side=Left
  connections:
  Solid/RConn1 -- ReferenceFrame/RConn1 -- F/RConn1

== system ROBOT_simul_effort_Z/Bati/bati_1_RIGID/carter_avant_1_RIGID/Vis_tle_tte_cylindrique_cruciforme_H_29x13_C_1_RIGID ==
  ReferenceFrame : sm_lib/Frames and Transforms/Reference Frame
  Solid : sm_lib/Body Elements/File Solid  ExtGeomFileName=/MATLAB Drive/Fichiers_Matlab_sujetA/Fichiers Matlab/STL/Vis a tole tete cylindrique cruciforme H 2-9x13 - C_Realiste_sldprt.STL  UnitType=Custom  ExtGeomFileUnits=mm  StepReaderType=HEX  ExportConvexHullGeometry=off  InertiaType=Custom  BasedOnType=Density  Density=1000  DensityUnits=kg/(m^3)  Mass=8.3821869835456372e-05  MassUnits=kg  CenterOfMass=[4.9478681581074904 0.00064910481891303923 -0.0013634218224953438]  CenterOfMassUnits=mm  MomentsOfInertia=[0.00016543197172893975 0.0014334630955093895 0.0014333390308476422]  MomentsOfInertiaUnits=kg*mm^2  ProductsOfInertia=[-5.4062904633677868e-09 -1.3111174919527308e-07 6.0713893531177014e-07]  ProductsOfInertiaUnits=kg*mm^2  GraphicType=FromGeometry  MarkerShape=Sphere  MarkerSize=10  GraphicVisPropType=SimpleVisualProperties  GraphicDiffuseColor=[0.75294117647058822 0.75294117647058822 0.75294117647058822]  GraphicOpacity=1  GraphicSpecularColor=[0.5 0.5 0.5 1.0]  GraphicAmbientColor=[0.15 0.15 0.15 1.0]  GraphicEmissiveColor=[0.0 0.0 0.0 1.0]  GraphicShininess=75  DoExposeReferenceFrame=on  SerializedFrames=<Frames/>
  F : PMIOPort  Side=Left
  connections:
  Solid/RConn1 -- ReferenceFrame/RConn1 -- F/RConn1

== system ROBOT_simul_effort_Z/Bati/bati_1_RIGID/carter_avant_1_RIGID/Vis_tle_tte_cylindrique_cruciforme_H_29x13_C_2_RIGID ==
  ReferenceFrame : sm_lib/Frames and Transforms/Reference Frame
  Solid : sm_lib/Body Elements/File Solid  ExtGeomFileName=/MATLAB Drive/Fichiers_Matlab_sujetA/Fichiers Matlab/STL/Vis a tole tete cylindrique cruciforme H 2-9x13 - C_Realiste_sldprt.STL  UnitType=Custom  ExtGeomFileUnits=mm  StepReaderType=HEX  ExportConvexHullGeometry=off  InertiaType=Custom  BasedOnType=Density  Density=1000  DensityUnits=kg/(m^3)  Mass=8.3821869835456372e-05  MassUnits=kg  CenterOfMass=[4.9478681581074904 0.00064910481891303923 -0.0013634218224953438]  CenterOfMassUnits=mm  MomentsOfInertia=[0.00016543197172893975 0.0014334630955093895 0.0014333390308476422]  MomentsOfInertiaUnits=kg*mm^2  ProductsOfInertia=[-5.4062904633677868e-09 -1.3111174919527308e-07 6.0713893531177014e-07]  ProductsOfInertiaUnits=kg*mm^2  GraphicType=FromGeometry  MarkerShape=Sphere  MarkerSize=10  GraphicVisPropType=SimpleVisualProperties  GraphicDiffuseColor=[0.75294117647058822 0.75294117647058822 0.75294117647058822]  GraphicOpacity=1  GraphicSpecularColor=[0.5 0.5 0.5 1.0]  GraphicAmbientColor=[0.15 0.15 0.15 1.0]  GraphicEmissiveColor=[0.0 0.0 0.0 1.0]  GraphicShininess=75  DoExposeReferenceFrame=on  SerializedFrames=<Frames/>
  F : PMIOPort  Side=Left
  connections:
  Solid/RConn1 -- ReferenceFrame/RConn1 -- F/RConn1

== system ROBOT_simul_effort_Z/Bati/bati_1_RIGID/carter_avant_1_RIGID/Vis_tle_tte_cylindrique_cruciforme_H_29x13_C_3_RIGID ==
  ReferenceFrame : sm_lib/Frames and Transforms/Reference Frame
  Solid : sm_lib/Body Elements/File Solid  ExtGeomFileName=/MATLAB Drive/Fichiers_Matlab_sujetA/Fichiers Matlab/STL/Vis a tole tete cylindrique cruciforme H 2-9x13 - C_Realiste_sldprt.STL  UnitType=Custom  ExtGeomFileUnits=mm  StepReaderType=HEX  ExportConvexHullGeometry=off  InertiaType=Custom  BasedOnType=Density  Density=1000  DensityUnits=kg/(m^3)  Mass=8.3821869835456372e-05  MassUnits=kg  CenterOfMass=[4.9478681581074904 0.00064910481891303923 -0.0013634218224953438]  CenterOfMassUnits=mm  MomentsOfInertia=[0.00016543197172893975 0.0014334630955093895 0.0014333390308476422]  MomentsOfInertiaUnits=kg*mm^2  ProductsOfInertia=[-5.4062904633677868e-09 -1.3111174919527308e-07 6.0713893531177014e-07]  ProductsOfInertiaUnits=kg*mm^2  GraphicType=FromGeometry  MarkerShape=Sphere  MarkerSize=10  GraphicVisPropType=SimpleVisualProperties  GraphicDiffuseColor=[0.75294117647058822 0.75294117647058822 0.75294117647058822]  GraphicOpacity=1  GraphicSpecularColor=[0.5 0.5 0.5 1.0]  GraphicAmbientColor=[0.15 0.15 0.15 1.0]  GraphicEmissiveColor=[0.0 0.0 0.0 1.0]  GraphicShininess=75  DoExposeReferenceFrame=on  SerializedFrames=<Frames/>
  F : PMIOPort  Side=Left
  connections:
  Solid/RConn1 -- ReferenceFrame/RConn1 -- F/RConn1

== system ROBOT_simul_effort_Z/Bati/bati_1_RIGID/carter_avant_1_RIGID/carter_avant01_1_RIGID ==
  ReferenceFrame : sm_lib/Frames and Transforms/Reference Frame
  Solid : sm_lib/Body Elements/File Solid  ExtGeomFileName=/MATLAB Drive/Fichiers_Matlab_sujetA/Fichiers Matlab/STL/carter avant01_Defaut_sldprt.STL  UnitType=Custom  ExtGeomFileUnits=mm  StepReaderType=HEX  ExportConvexHullGeometry=off  InertiaType=Custom  BasedOnType=Density  Density=1000  DensityUnits=kg/(m^3)  Mass=0.037834193553807655  MassUnits=kg  CenterOfMass=[-1.2122189045492688 175.43270841498617 61.584507438849911]  CenterOfMassUnits=mm  MomentsOfInertia=[56.040868119625912 128.12274252763086 98.880664351206846]  MomentsOfInertiaUnits=kg*mm^2  ProductsOfInertia=[17.771132404811137 -0.72051019684540141 0.93869411089982313]  ProductsOfInertiaUnits=kg*mm^2  GraphicType=FromGeometry  MarkerShape=Sphere  MarkerSize=10  GraphicVisPropType=SimpleVisualProperties  GraphicDiffuseColor=[1.0 1.0 1.0]  GraphicOpacity=0  GraphicSpecularColor=[0.5 0.5 0.5 1.0]  GraphicAmbientColor=[0.15 0.15 0.15 1.0]  GraphicEmissiveColor=[0.0 0.0 0.0 1.0]  GraphicShininess=75  DoExposeReferenceFrame=on  SerializedFrames=<Frames/>
  F : PMIOPort  Side=Left
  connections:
  Solid/RConn1 -- ReferenceFrame/RConn1 -- F/RConn1

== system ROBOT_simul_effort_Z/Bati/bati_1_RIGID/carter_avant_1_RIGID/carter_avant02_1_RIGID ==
  ReferenceFrame : sm_lib/Frames and Transforms/Reference Frame
  Solid : sm_lib/Body Elements/File Solid  ExtGeomFileName=/MATLAB Drive/Fichiers_Matlab_sujetA/Fichiers Matlab/STL/carter avant02_Defaut_sldprt.STL  UnitType=Custom  ExtGeomFileUnits=mm  StepReaderType=HEX  ExportConvexHullGeometry=off  InertiaType=Custom  BasedOnType=Density  Density=1000  DensityUnits=kg/(m^3)  Mass=0.04003612730019273  MassUnits=kg  CenterOfMass=[-5.5302874316411099 176.12322006317407 58.915594608725293]  CenterOfMassUnits=mm  MomentsOfInertia=[61.433722156029233 146.06754836858084 112.39719793476846]  MomentsOfInertiaUnits=kg*mm^2  ProductsOfInertia=[19.11954141989958 -8.6708453597958446 2.8769308330981094]  ProductsOfInertiaUnits=kg*mm^2  GraphicType=FromGeometry  MarkerShape=Sphere  MarkerSize=10  GraphicVisPropType=SimpleVisualProperties  GraphicDiffuseColor=[1.0 1.0 1.0]  GraphicOpacity=1  GraphicSpecularColor=[0.5 0.5 0.5 1.0]  GraphicAmbientColor=[0.15 0.15 0.15 1.0]  GraphicEmissiveColor=[0.0 0.0 0.0 1.0]  GraphicShininess=75  DoExposeReferenceFrame=on  SerializedFrames=<Frames/>
  F : PMIOPort  Side=Left
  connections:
  Solid/RConn1 -- ReferenceFrame/RConn1 -- F/RConn1

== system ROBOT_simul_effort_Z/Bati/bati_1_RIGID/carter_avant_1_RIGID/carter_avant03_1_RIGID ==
  ReferenceFrame : sm_lib/Frames and Transforms/Reference Frame
  Solid : sm_lib/Body Elements/File Solid  ExtGeomFileName=/MATLAB Drive/Fichiers_Matlab_sujetA/Fichiers Matlab/STL/carter avant03_Defaut_sldprt.STL  UnitType=Custom  ExtGeomFileUnits=mm  StepReaderType=HEX  ExportConvexHullGeometry=off  InertiaType=Custom  BasedOnType=Density  Density=1000  DensityUnits=kg/(m^3)  Mass=0.040033100851173897  MassUnits=kg  CenterOfMass=[3.2488267644133511 176.1208864671479 58.924212973359204]  CenterOfMassUnits=mm  MomentsOfInertia=[61.470691722682709 146.87719070674399 113.21967982116205]  MomentsOfInertiaUnits=kg*mm^2  ProductsOfInertia=[19.138525158618911 7.4477910669264711 -1.062715139795626]  ProductsOfInertiaUnits=kg*mm^2  GraphicType=FromGeometry  MarkerShape=Sphere  MarkerSize=10  GraphicVisPropType=SimpleVisualProperties  GraphicDiffuseColor=[1.0 1.0 1.0]  GraphicOpacity=1  GraphicSpecularColor=[0.5 0.5 0.5 1.0]  GraphicAmbientColor=[0.15 0.15 0.15 1.0]  GraphicEmissiveColor=[0.0 0.0 0.0 1.0]  GraphicShininess=75  DoExposeReferenceFrame=on  SerializedFrames=<Frames/>
  F : PMIOPort  Side=Left
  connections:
  Solid/RConn1 -- ReferenceFrame/RConn1 -- F/RConn1

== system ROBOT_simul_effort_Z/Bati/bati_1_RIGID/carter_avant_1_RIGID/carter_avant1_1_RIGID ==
  ReferenceFrame : sm_lib/Frames and Transforms/Reference Frame
  Solid : sm_lib/Body Elements/File Solid  ExtGeomFileName=/MATLAB Drive/Fichiers_Matlab_sujetA/Fichiers Matlab/STL/carter avant1_Defaut_sldprt.STL  UnitType=Custom  ExtGeomFileUnits=mm  StepReaderType=HEX  ExportConvexHullGeometry=off  InertiaType=Custom  BasedOnType=Density  Density=1000  DensityUnits=kg/(m^3)  Mass=0.0068977261305129805  MassUnits=kg  CenterOfMass=[0.013428833188053345 115.01841988578165 104.87566191405597]  CenterOfMassUnits=mm  MomentsOfInertia=[2.0334532747861105 2.0241587370426406 3.5278352594861393]  MomentsOfInertiaUnits=kg*mm^2  ProductsOfInertia=[-0.0020444395438733434 -2.1966864026409714e-05 -0.00053475799446389791]  ProductsOfInertiaUnits=kg*mm^2  GraphicType=FromGeometry  MarkerShape=Sphere  MarkerSize=10  GraphicVisPropType=SimpleVisualProperties  GraphicDiffuseColor=[0.792156862745098 0.81960784313725488 0.93333333333333335]  GraphicOpacity=1  GraphicSpecularColor=[0.5 0.5 0.5 1.0]  GraphicAmbientColor=[0.15 0.15 0.15 1.0]  GraphicEmissiveColor=[0.0 0.0 0.0 1.0]  GraphicShininess=75  DoExposeReferenceFrame=on  SerializedFrames=<Frames/>
  F : PMIOPort  Side=Left
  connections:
  Solid/RConn1 -- ReferenceFrame/RConn1 -- F/RConn1

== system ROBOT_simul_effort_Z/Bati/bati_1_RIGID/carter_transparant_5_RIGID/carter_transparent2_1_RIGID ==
  ReferenceFrame : sm_lib/Frames and Transforms/Reference Frame
  Solid : sm_lib/Body Elements/File Solid  ExtGeomFileName=/MATLAB Drive/Fichiers_Matlab_sujetA/Fichiers Matlab/STL/carter transparent2_Defaut_sldprt.STL  UnitType=Custom  ExtGeomFileUnits=mm  StepReaderType=HEX  ExportConvexHullGeometry=off  InertiaType=Custom  BasedOnType=Density  Density=1000  DensityUnits=kg/(m^3)  Mass=0.09082975360372901  MassUnits=kg  CenterOfMass=[2.3301793536057773 71.397337965148168 56.68444733144738]  CenterOfMassUnits=mm  MomentsOfInertia=[150.08149768370154 164.27950343498205 187.86724715852677]  MomentsOfInertiaUnits=kg*mm^2  ProductsOfInertia=[-19.998213794105411 -3.3083924529632989 0.84436764044313561]  ProductsOfInertiaUnits=kg*mm^2  GraphicType=FromGeometry  MarkerShape=Sphere  MarkerSize=10  GraphicVisPropType=SimpleVisualProperties  GraphicDiffuseColor=[0.792156862745098 0.81960784313725488 0.93333333333333335]  GraphicOpacity=1  GraphicSpecularColor=[0.5 0.5 0.5 1.0]  GraphicAmbientColor=[0.15 0.15 0.15 1.0]  GraphicEmissiveColor=[0.0 0.0 0.0 1.0]  GraphicShininess=75  DoExposeReferenceFrame=on  SerializedFrames=<Frames/>
  F : PMIOPort  Side=Left
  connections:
  Solid/RConn1 -- ReferenceFrame/RConn1 -- F/RConn1
